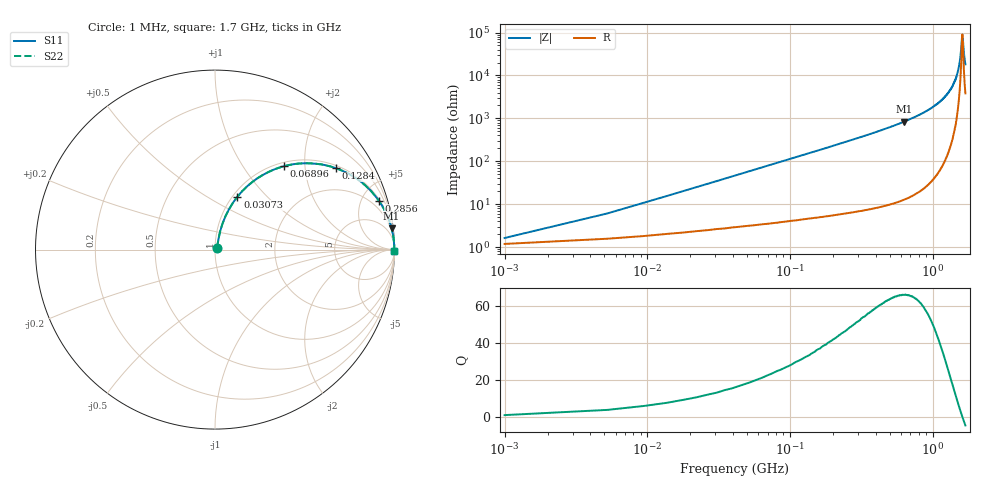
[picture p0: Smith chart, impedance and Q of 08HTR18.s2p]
! Coilcraft 0805HT-R18 Chip Inductor
! 6 August 2004
# MHZ S MA R 50
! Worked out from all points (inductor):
!   401 points, 1 MHz to 1.7 GHz, reference 50 ohm
!   read as one part in series: L = 179 nH near 9.495 MHz
!   highest Q = 65.8 at 629.6 MHz (marker M1), where L = 210 nH
!   self-resonance near 1.615 GHz
!   S11 on the Smith chart (normalised r, x): 1 MHz: 1.02, +0.02; 30.73 MHz: 1.05, +0.69; 68.96 MHz: 1.07, +1.55; 128.4 MHz: 1.09, +2.91; 285.6 MHz: 1.14, +6.63; 1.7 GHz: open
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1  0.016 43.1  0.988 -0.6  0.988 -0.6  0.016 43.1
13.743  0.151 73.9  0.969 -8.6  0.969 -8.6  0.151 73.9
22.237  0.238 70.9  0.949 -13.7  0.949 -13.7  0.238 70.9
30.732  0.32 67.0  0.923 -18.6  0.923 -18.6  0.32 67.0
47.722  0.463 59.2  0.86 -27.5  0.86 -27.5  0.463 59.2
68.96  0.601 50.5  0.773 -36.9  0.773 -36.9  0.601 50.5
128.425  0.812 33.9  0.559 -54.3  0.559 -54.3  0.812 33.9
192.138  0.902 24.3  0.411 -64.3  0.411 -64.3  0.902 24.3
285.583  0.952 16.7  0.287 -72.2  0.287 -72.2  0.952 16.7
570.165  0.989 7.8  0.135 -81.4  0.135 -81.4  0.989 7.8
629.63  0.991 6.8  0.119 -82.3  0.119 -82.3  0.991 6.8
850.5  0.996 4.3  0.075 -84.7  0.075 -84.7  0.996 4.3
1135.082  0.998 2.3  0.04 -86.2  0.04 -86.2  0.998 2.3
1287.992  0.999 1.4  0.025 -86.3  0.025 -86.3  0.999 1.4
1419.665  0.999 0.8  0.014 -85.1  0.014 -85.1  0.999 0.8
1479.13  0.999 0.6  0.009974 -83.4  0.009974 -83.4  0.999 0.6
1538.595  0.999 0.3  0.005686 -78.8  0.005686 -78.8  0.999 0.3
1572.575  0.999 0.2  0.003366 -71.0  0.003366 -71.0  0.999 0.2
1610.802  0.999 0.0  0.001234 -26.5  0.001234 -26.5  0.999 0.0
1619.297  0.999 -0.0  0.001108 1.3  0.001108 1.3  0.999 -0.0
1666.02  0.999 -0.2  0.003345 70.0  0.003345 70.0  0.999 -0.2
1700  0.999 -0.3  0.005486 77.5  0.005486 77.5  0.999 -0.3
